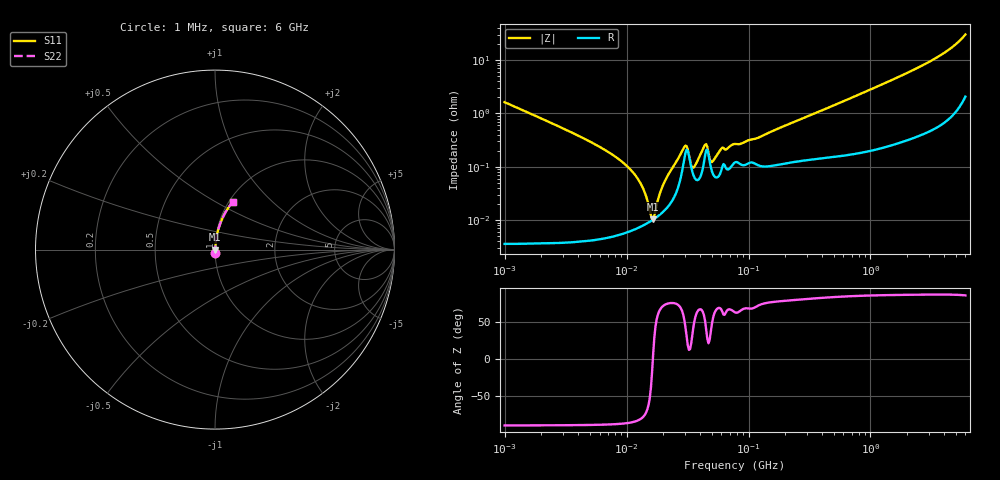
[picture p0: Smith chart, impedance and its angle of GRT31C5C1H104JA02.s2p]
!Murata Part Number: GRT31C5C1H104JA02
!These Parameters are Measured in Series Mode Connection
!Data Generated on Jun 19, 2026
!  o--ll--o
!Port1  Port2
!  o------o
!Operation Temp=25[degC], DC Bias Voltage=0[V]
!Freq. Start=1000[kHz] Stop=6[GHz] 401[Steps]
# Hz S RI R 50
!Freq.(Hz) S11(Real) S11(Imag) S21(Real) S21(Imag) S12(Real) S12(Imag) S22(Real) S22(Imag)
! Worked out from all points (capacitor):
!   401 points, 1 MHz to 6 GHz, reference 50 ohm
!   read as one part in series: C = 97.4 nF near 1.044 MHz
!   lowest |Z| = 10.4 mohm at 16.54 MHz (marker M1)
!   series resonance near 16.43 MHz, so ESL is about 960 pH
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1000000  0.000301 -0.0163  0.9997 0.0163  0.9997 0.0163  0.000301 -0.0163
4293785  5.25e-05 -0.00356  0.9999 0.00356  0.9999 0.00356  5.25e-05 -0.00356
7558231  5.17e-05 -0.00172  0.9999 0.00172  0.9999 0.00172  5.17e-05 -0.00172
1.093935e7  6.4e-05 -0.000852  0.9999 0.000852  0.9999 0.000852  6.4e-05 -0.000852
1.330454e7  7.74e-05 -0.00044  0.9999 0.00044  0.9999 0.00044  7.74e-05 -0.00044
1.583299e7  9.64e-05 -7.82e-05  0.9999 7.82e-05  0.9999 7.82e-05  9.64e-05 -7.82e-05
1.653689e7  0.000103 1.38e-05  0.9999 -1.38e-05  0.9999 -1.38e-05  0.000103 1.38e-05
1.843659e7  0.000123 0.000252  0.9999 -0.000252  0.9999 -0.000252  0.000123 0.000252
2.100646e7  0.000162 0.000566  0.9998 -0.000566  0.9998 -0.000566  0.000162 0.000566
2.974945e7  0.00142 0.00188  0.9986 -0.00188  0.9986 -0.00188  0.00142 0.00188
3.107204e7  0.0021 0.00122  0.9979 -0.00122  0.9979 -0.00122  0.0021 0.00122
3.389622e7  0.000989 0.000388  0.999 -0.000388  0.999 -0.000388  0.000989 0.000388
3.540316e7  0.00069 0.000673  0.9993 -0.000673  0.9993 -0.000673  0.00069 0.000673
4.400437e7  0.00161 0.00203  0.9984 -0.00203  0.9984 -0.00203  0.00161 0.00203
5.013812e7  0.000821 0.000907  0.9992 -0.000907  0.9992 -0.000907  0.000821 0.000907
5.966657e7  0.000845 0.00201  0.9992 -0.00201  0.9992 -0.00201  0.000845 0.00201
7.745967e7  0.00122 0.00239  0.9988 -0.00239  0.9988 -0.00239  0.00122 0.00239
1.196694e8  0.00108 0.00333  0.9989 -0.00333  0.9989 -0.00333  0.00108 0.00333
3.325952e8  0.00146 0.00946  0.9985 -0.00946  0.9985 -0.00946  0.00146 0.00946
1.428092e9  0.00406 0.04  0.9959 -0.04  0.9959 -0.04  0.00406 0.04
3.5601e9  0.0182 0.1117  0.9818 -0.1117  0.9818 -0.1117  0.0182 0.1117
6e9  0.0989 0.2662  0.9011 -0.2662  0.9011 -0.2662  0.0989 0.2662
